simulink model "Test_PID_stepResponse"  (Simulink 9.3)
settings: Solver=VariableStepAuto  StartTime=0.0  StopTime=10.0  RelTol=1e-3
InitFcn:
  | Tstep=0.000050;
  | Tparam=0.002;
  | Tinit=0.010;
  | stimuli_path_Test_PID='test/Smlk/+Test_LibVishia_Ctrl/+stimuli/stimuli_TestCtrl.m'
libraries: libVishia_Inspc x5, libVishia_CtrlSfn x4, libVishia_Ctrl x3

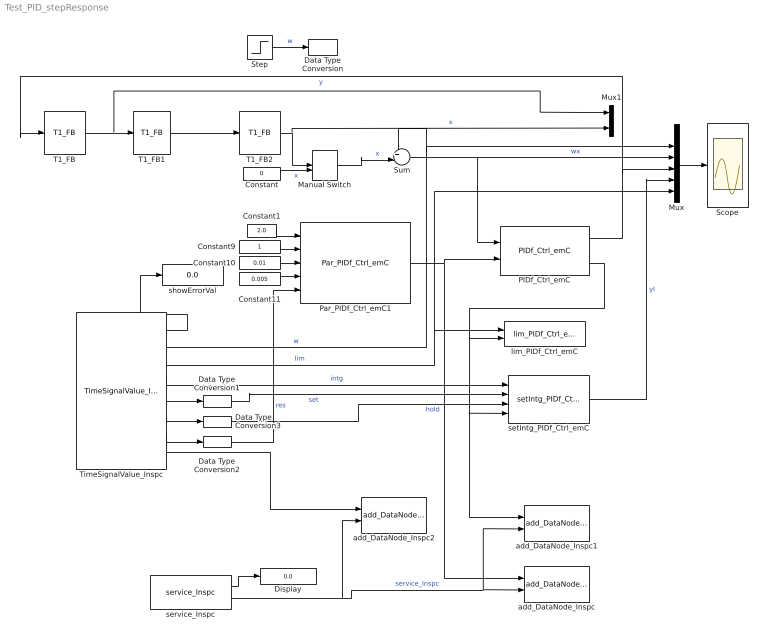
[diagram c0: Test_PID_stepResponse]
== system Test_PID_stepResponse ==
  Constant : Constant  Value=0  OutDataTypeStr=single
  Constant1 : Constant  Value=2.0  OutDataTypeStr=single  SampleTime=-1
  Constant10 : Constant  Value=0.01  OutDataTypeStr=single  SampleTime=-1
  Constant11 : Constant  Value=0.005  OutDataTypeStr=single  SampleTime=-1
  Constant9 : Constant  OutDataTypeStr=single  SampleTime=-1
  Data Type Conversion : DataTypeConversion  OutDataTypeStr=single
  Data Type Conversion1 : DataTypeConversion  OutDataTypeStr=boolean
  Data Type Conversion2 : DataTypeConversion  OutDataTypeStr=boolean
  Data Type Conversion3 : DataTypeConversion  OutDataTypeStr=boolean
  Display : Display
  Manual Switch : ManualSwitch
  Mux : Mux  Inputs=6
  Mux1 : Mux  Inputs=3
  PIDf_Ctrl_emC : libVishia_CtrlSfn/PIDf_Ctrl_emC  Tstep=Tstep
  Par_PIDf_Ctrl_emC1 : libVishia_CtrlSfn/Par_PIDf_Ctrl_emC  Tparam=Tparam  Tctrl=Tstep  yMax=10  openLoop=0
  Scope : Scope
  Step : Step  SampleTime=0
  Sum : Sum  Inputs=+-|
  T1_FB : libVishia_Ctrl/T1_FB  T1=0.1  y0=0  Tstep=Tstep
  T1_FB1 : libVishia_Ctrl/T1_FB  T1=0.03  y0=0  Tstep=Tstep
  T1_FB2 : libVishia_Ctrl/T1_FB  T1=0.03  y0=0  Tstep=Tstep
  TimeSignalValue_Inspc : libVishia_Inspc/TimeSignalValue_Inspc  Description=|  Tstep=Tstep  filepath=stimuli_path_Test_PID  nameRefl='test'  nrofStimuli=25  varDef=|
      | A combined stimuli and inspector function block.
      | Stimuli file path: file contains stimuli in form:
      |   %time:0: stimuli.namex = 5000.0, stimuli.namey = 50.0 -10; 
      | Name in reflection-tree: Name of this function block for stimuli and inspector access
      | name1..12: output type and name, base type is single always.
      | C2:namexy  A complex array of 2 elements
      | 6:namexy An array of 6 elements (max).
      | C:namexy  A 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
      | x: F;
      | lim: F;
      | intg: F;
      | set: F;
      | hold: F;
      | res: F;
  add_DataNode_Inspc : libVishia_Inspc/add_DataNode_Inspc  name1Refl='main'  name2Refl='_PIDparam'
  add_DataNode_Inspc1 : libVishia_Inspc/add_DataNode_Inspc  name1Refl='main'  name2Refl='_PID'
  add_DataNode_Inspc2 : libVishia_Inspc/add_DataNode_Inspc  name1Refl='test'  name2Refl=''
  lim_PIDf_Ctrl_emC : libVishia_CtrlSfn/lim_PIDf_Ctrl_emC
  service_Inspc : libVishia_Inspc/service_Inspc  Tstep=Tstep  IpPort='UDP:0.0.0.0:60094'
  setIntg_PIDf_Ctrl_emC : libVishia_CtrlSfn/setIntg_PIDf_Ctrl_emC
  showErrorVal : Display
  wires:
  Step/1 -> Data Type Conversion/1  "w"
  Manual Switch/1 -> Sum/2  "x"
  Constant9/1 -> Par_PIDf_Ctrl_emC1/2
  Constant10/1 -> Par_PIDf_Ctrl_emC1/3
  Constant1/1 -> Par_PIDf_Ctrl_emC1/1
  Par_PIDf_Ctrl_emC1/1 -> PIDf_Ctrl_emC/2, add_DataNode_Inspc/1
  Constant11/1 -> Par_PIDf_Ctrl_emC1/4
  Sum/1 -> Mux/3, PIDf_Ctrl_emC/1  "wx"
  TimeSignalValue_Inspc/2 -> Sum/1, Mux/2  "w"
  Mux/1 -> Scope/1
  PIDf_Ctrl_emC/1 -> T1_FB/1, Mux/4  "y"
  service_Inspc/2 -> add_DataNode_Inspc2/2, add_DataNode_Inspc1/2, add_DataNode_Inspc/2  "service_Inspc"
  service_Inspc/1 -> Display/1
  PIDf_Ctrl_emC/3 -> lim_PIDf_Ctrl_emC/2, setIntg_PIDf_Ctrl_emC/4, add_DataNode_Inspc1/1
  T1_FB/2 -> Mux1/1, T1_FB1/1
  T1_FB1/2 -> T1_FB2/1
  T1_FB2/2 -> Manual Switch/1, Mux1/3  "x"
  Constant/1 -> Manual Switch/2  "x"
  TimeSignalValue_Inspc/1 -> showErrorVal/1
  TimeSignalValue_Inspc/3 -> Mux/6, lim_PIDf_Ctrl_emC/1  "lim"
  TimeSignalValue_Inspc/4 -> setIntg_PIDf_Ctrl_emC/1  "intg"
  TimeSignalValue_Inspc/5 -> Data Type Conversion1/1
  Data Type Conversion1/1 -> setIntg_PIDf_Ctrl_emC/2  "set"
  TimeSignalValue_Inspc/8 -> add_DataNode_Inspc2/1
  TimeSignalValue_Inspc/7 -> Data Type Conversion2/1
  Data Type Conversion2/1 -> Par_PIDf_Ctrl_emC1/5  "res"
  TimeSignalValue_Inspc/6 -> Data Type Conversion3/1
  Data Type Conversion3/1 -> setIntg_PIDf_Ctrl_emC/3  "hold"
  Mux1/1 -> ?
  setIntg_PIDf_Ctrl_emC/1 -> Mux/5  "yI"
